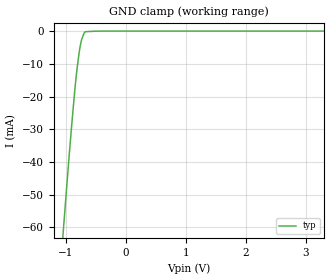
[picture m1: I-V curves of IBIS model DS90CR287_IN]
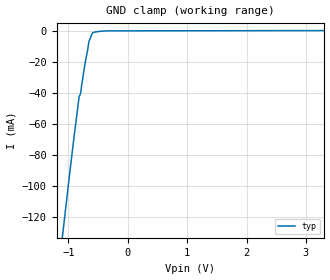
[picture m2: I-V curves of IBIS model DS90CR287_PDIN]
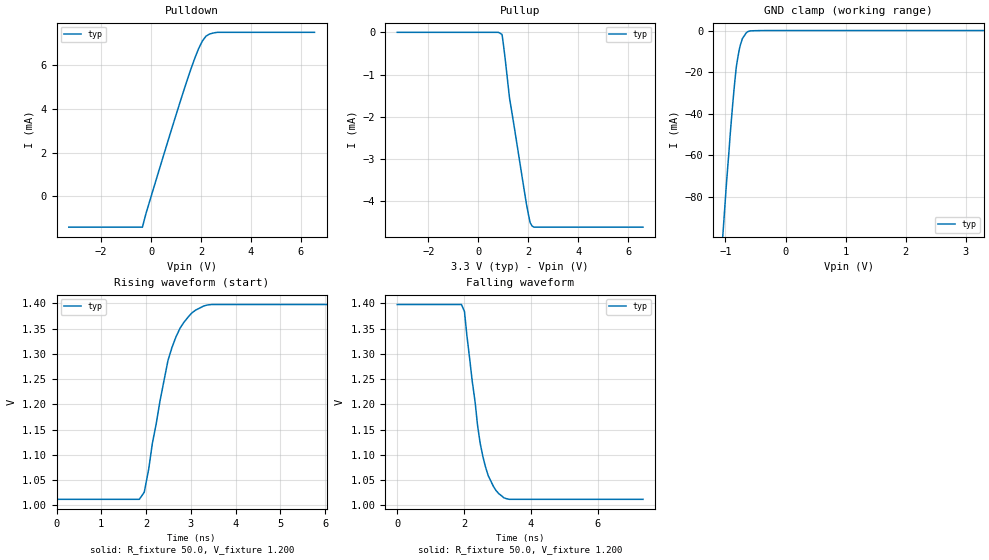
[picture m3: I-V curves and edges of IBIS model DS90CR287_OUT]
|   National Semiconductor Corporation
|   Interface Products Group
|   IBIS Model of DS90CR287MTD
|   High Speed Link Transmitter
|   56L TSSOP
[IBIS Ver]   3.2
[Comment char]  |_char
[File name]   ds90cr287.ibs
[File Rev]   1.4
[Date]   9/26/03
[Source]   File originated at National Semiconductor Corporation.
   Interface Group/Analog Division. All data based on
   Empirical Measurements(Bench).
[Notes]   File created by DT.
   Revision 1.0: The original model.
   Revision 1.1: Modified driver output pulldown
   and pullup to ensure no double
   counting of clamp current.
   Revision 1.2: Corrected ground and power clamp data.
   Revision 1.3: Changed Vdiff from .1 to 0 in pin mapping
   Changed Vref from 0 to 1.2 in V/T data
   Commented out c_fixutre in V/T data
   Revision 1.4: Modified pullup, pulldown,
   rising and falling waveform data;
[Disclaimer]
(C) Copyright National Semiconductor Corporation 2000
   All rights reserved
   National Semiconductor Corporation hereby grants
the user of this IBIS model a non-exclusive, nontransferable
license to use this IBIS model under the following terms.
Before using this IBIS model, the user should read this
license.  If the user does not accept these terms, the
IBIS model should be returned to National within 30 days.
   The user is granted this license only to use the
IBIS model and is not granted rights to sell, load, rent,
lease or license the IBIS model in whole or in part, or in
modified form to anyone other than user. User may modify
the IBIS model to suit its specific applications but rights
to derivative works and such modifications shall belong to
National.
   This IBIS model is provided on an "AS IS" basis and
National makes absolutely no warranty with respect to the
information contained herein. NATIONAL DISCLAIMS AND CUSTOMER
WAIVES ALL WARRANTIES, EXPRESS OR IMPLIED, INCLUDING
WARRANTIES OF MERCHANTABILITY OR FITNESS FOR A PARTICULAR
PURPOSE. The entire risk as to quality and performance is
with the Customer. ACCORDINGLY, IN NO EVENT SHALL THE
COMPANY BE LIABLE FOR ANY DAMAGES, WHETHER IN CONTRACT OR
TORT,INCLUDING ANY LOST PROFITS OR OTHER INCIDENTAL,
CONSEQUENTIAL, EXEMPLARY, OR PUNITIVE DAMAGES ARISING OUT
OF THE USE OR APPLICATION OF THE IBIS model provided in
this package. Further, National reserves the right to make
changes without notice to any product herein to improve
reliability, function, or design. National does not convey
any license under patent rights or any other intellectual
property rights, including those of third parties.
   National is not obligated to provide maintenance or support
for the licensed IBIS model.
Contact National at ATTN:INTERFACE APPLICATIONS/IBIS MODELS.
2900 Semiconductor Drive, M/S A2595, Santa Clara, CA 95052-8090
[Copyright]   Copyright 2000, National Semiconductor, All Rights Reserved
[Component]   DS90CR287MTD
[Manufacturer]  National Semiconductor Corp
[Package]
|   typ   min   max
R_pkg   61.4m   NA   NA
L_pkg   1.758nH   NA   NA
C_pkg   0.075pF   NA   NA
[Pin]   signal_name   model_name   R_pin   L_pin   C_pin
1   VCC   POWER   90.0m   3.077n   0.122p
2   TxIN5   DS90CR287_IN   90.0m   2.704n   0.107p
3   TxIN6   DS90CR287_IN   90.0m   2.405n   0.106p
4   TxIN7   DS90CR287_IN   70.0m   2.105n   0.096p
5   GND   GND   70.0m   1.874n   0.080p
6   TxIN8   DS90CR287_IN   60.0m   1.619n   0.071p
7   TxIN9   DS90CR287_IN   60.0m   1.414n   0.068p
8   TxIN10   DS90CR287_IN   60.0m   1.405n   0.068p
9   Vcc   POWER   50.0m   1.407n   0.055p
10   TxIN11   DS90CR287_IN   50.0m   1.396n   0.055p
11   TxIN12   DS90CR287_IN   50.0m   1.365n   0.055p
12   TxIN13   DS90CR287_IN   50.0m   1.318n   0.055p
13   GND   GND   40.0m   1.277n   0.057p
14   TxIN14   DS90CR287_IN   30.0m   1.249n   0.061p
15   TxIN15   DS90CR287_IN   30.0m   1.249n   0.061p
16   TxIN16   DS90CR287_IN   40.0m   1.277n   0.057p
17   Vcc   POWER   50.0m   1.318n   0.055p
18   TxIN17   DS90CR287_IN   50.0m   1.365n   0.055p
19   TxIN18   DS90CR287_IN   50.0m   1.396n   0.055p
20   TxIN19   DS90CR287_IN   50.0m   1.407n   0.055p
21   GND   GND   60.0m   1.405n   0.068p
22   TxIN20   DS90CR287_IN   60.0m   1.414n   0.068p
23   TxIN21   DS90CR287_IN   60.0m   1.619n   0.071p
24   TxIN22   DS90CR287_IN   70.0m   1.874n   0.080p
25   TxIN23   DS90CR287_IN   70.0m   2.105n   0.096p
26   Vcc   POWER   90.0m   2.405n   0.106p
27   TxIN24   DS90CR287_IN   90.0m   2.704n   0.107p
28   TxIN25   DS90CR287_IN   90.0m   3.077n   0.122p
29   GND   GND   90.0m   3.077n   0.122p
30   TxIN26   DS90CR287_IN   90.0m   2.704n   0.107p
31   TxCLKIN   DS90CR287_IN   90.0m   2.405n   0.106p
32   PWRDWN*   DS90CR287_PDIN   70.0m   2.105n   0.096p
33   PLLGND   GND   70.0m   1.874n   0.080p
34   PLLVCC   POWER   60.0m   1.619n   0.071p
35   PLLGND   GND   60.0m   1.414n   0.068p
36   LVDSGND   GND   60.0m   1.405n   0.068p
37   TxOUT3+   DS90CR287_OUT   50.0m   1.407n   0.055p
38   TxOUT3-   DS90CR287_OUT   50.0m   1.396n   0.055p
39   TxCLKOUT   DS90CR287_OUT   50.0m   1.365n   0.055p
40   TxCLKOUT   DS90CR287_OUT   50.0m   1.318n   0.055p
41   TxOUT2+   DS90CR287_OUT   40.0m   1.277n   0.057p
42   TxOUT2-   DS90CR287_OUT   30.0m   1.249n   0.061p
43   LVDSGND   GND   30.0m   1.249n   0.061p
44   LVDSVCC   POWER   40.0m   1.277n   0.057p
45   TxOUT1+   DS90CR287_OUT   50.0m   1.318n   0.055p
46   TxOUT1-   DS90CR287_OUT   50.0m   1.365n   0.055p
47   TxOUT0+   DS90CR287_OUT   50.0m   1.396n   0.055p
48   TxOUT0-   DS90CR287_OUT   50.0m   1.407n   0.055p
49   LVDSGND   GND   60.0m   1.405n   0.068p
50   TxIN27   DS90CR287_IN   60.0m   1.414n   0.068p
51   TxIN0   DS90CR287_IN   60.0m   1.619n   0.071p
52   TxIN1   DS90CR287_IN   70.0m   1.874n   0.080p
53   GND   GND   70.0m   2.105n   0.096p
54   TxIN2   DS90CR287_IN   90.0m   2.405n   0.106p
55   TxIN3   DS90CR287_IN   90.0m   2.704n   0.107p
56   TxIN4   DS90CR287_IN   90.0m   3.077n   0.122p
[Diff_pin]   inv_pin   vdiff   tdelay_typ   tdelay_min   tdelay_max
| The '+' pin is Diff_pin and the '-' pin is the inv_pin
37   38   0.0   0   0   0
39   40   0.0   0   0   0
41   42   0.0   0   0   0
45   46   0.0   0   0   0
47   48   0.0   0   0   0
| Models and submodels in the file (3): DS90CR287_IN (Input), DS90CR287_PDIN (Input), DS90CR287_OUT (3-state)
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|   Driver Input  MODEL
[Model]   DS90CR287_IN
Model_type   Input
|Signals   TxIN0 ~ TxIN27
Vinh = 2.0
Vinl = 0.8
|   typ   min   max
C_comp   5.910pF   NA   NA
|   typ   min   max
[Temperature Range]   25.0   NA   NA
[Voltage range]   3.3V   3.0V   3.6V
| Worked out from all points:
|   GND clamp passes 1 mA (typ) near -0.70 V on its own axis
[Power_clamp]
| Note that the[POWER_clamp]voltage table is referenced to Vcc
| and is calculated using Vtable=Vcc - Vmeasured.
|Voltage   I(typ)   I(min)   I(max)
-3V       0A         NA         NA
3V        0A         NA         NA
[GND_clamp]
|Voltage   I(typ)   I(min)   I(max)
-3.3V     -594.1mA   NA         NA
-1.001V   -51.39mA   NA         NA
-941.2mV  -37.29mA   NA         NA
-899.9mV  -28.27mA   NA         NA
-859.6mV  -19.87mA   NA         NA
-818.3mV  -12.37mA   NA         NA
-776.9mV  -6.424mA   NA         NA
-756.3mV  -4.202mA   NA         NA
-736.1mV  -2.573mA   NA         NA
-717mV    -1.615mA   NA         NA
-675.2mV  -194.8uA   NA         NA
3.3V      524nA      NA         NA
|   Driver PWRDWN* Input  MODEL
[Model]   DS90CR287_PDIN
Model_type   Input
|Signals   PWRDWN*
Vinh = 2.0
Vinl = 0.8
|   typ   min   max
C_comp   5.843pF   NA   NA
|   typ   min   max
[Temperature Range]   25.0   NA   NA
[Voltage range]   3.3V   3.0V   3.6V
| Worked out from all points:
|   GND clamp passes 1 mA (typ) near -0.57 V on its own axis
[Power_clamp]
| Note that the[POWER_clamp]voltage table is referenced to Vcc
| and is calculated using Vtable=Vcc - Vmeasured.
|Voltage   I(typ)   I(min)   I(max)
-3V       0A         NA         NA
3V        0A         NA         NA
[GND_clamp]
|Voltage   I(typ)   I(min)   I(max)
-3.3V     -863.2mA   NA         NA
-999.7mV  -98.78mA   NA         NA
-918.6mV  -72.42mA   NA         NA
-819.7mV  -42.41mA   NA         NA
-796.1mV  -40.44mA   NA         NA
-776.9mV  -35.09mA   NA         NA
-735.6mV  -24.85mA   NA         NA
-674.7mV  -11.91mA   NA         NA
-655mV    -6.957mA   NA         NA
-592.5mV  -1.248mA   NA         NA
-306.8mV  -9.428uA   NA         NA
3.3V      172.6uA    NA         NA
|   Driver Output  MODEL
[Model]   DS90CR287_OUT
Model_type   3-state
| Signals   TxOUT0 ~ TxOUT3; TxCLKOUT
Vmeas = 1.2V   |This is 0.0v differential on output
Cref = 5pF   |Timing specification test load capacitance value
Rref = 50   |Note: 100 Ohm between the two driver outputs
Vref = 1.2   |Timing specification test load voltage; GND
| variable   typ   min   max
C_comp   6.704pF   NA   NA
|   typ   min   max
[Temperature Range]   25.0   NA   NA
[Voltage range]   3.3V   3.0V   3.6V
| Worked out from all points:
|   slope of the pulldown table from 0 to 0.495 V, typ, clamps not added: 266 ohm
|   GND clamp passes 1 mA (typ) near -0.65 V on its own axis
|   rising waveform, R_fixture 50.0, V_fixture 1.200: 20-80 % time 526ps typ, NA min, NA max; typ from 1.01 V to 1.4 V
|   falling waveform, R_fixture 50.0, V_fixture 1.200: 20-80 % time 479ps typ, NA min, NA max; typ from 1.4 V to 1.01 V
[Pulldown]
| Voltage   I(typ)   I(min)   I(max)
-3.3V     -1.408mA   NA         NA
-350mV    -1.408mA   NA         NA
-200mV    -758uA     NA         NA
475mV     1.786mA    NA         NA
1.45V     5.331mA    NA         NA
1.75V     6.312mA    NA         NA
1.9V      6.74mA     NA         NA
2.05V     7.09mA     NA         NA
2.2V      7.321mA    NA         NA
2.35V     7.422mA    NA         NA
2.65V     7.496mA    NA         NA
6.55V     7.496mA    NA         NA
[Pullup]
| Note that the[Pullup]voltage table is referenced to Vcc
| and is calculated using Vtable=Vcc - Vmeasured.
|Voltage   I(typ)   I(min)   I(max)
-3.25V    0A         NA         NA
800mV     -600nA     NA         NA
950mV     -51.4uA    NA         NA
1.025V    -380.3uA   NA         NA
1.1V      -755.3uA   NA         NA
1.25V     -1.556mA   NA         NA
1.4V      -2.095mA   NA         NA
1.925V    -4.051mA   NA         NA
2.075V    -4.497mA   NA         NA
2.15V     -4.577mA   NA         NA
2.225V    -4.607mA   NA         NA
6.6V      -4.607mA   NA         NA
[GND_clamp]
| Outputs in Tri-state.
| Voltage   I(typ)   I(min)   I(max)
-3.3V     -1.034A    NA         NA
-1.001V   -81.02mA   NA         NA
-983mV    -73.48mA   NA         NA
-921.5mV  -50.22mA   NA         NA
-900.9mV  -42.95mA   NA         NA
-859.6mV  -29.11mA   NA         NA
-819.2mV  -17.54mA   NA         NA
-767.2mV  -8.785mA   NA         NA
-719.4mV  -3.945mA   NA         NA
-634.3mV  -657.5uA   NA         NA
-347.7mV  -11.87uA   NA         NA
3.3V      524nA      NA         NA
[POWER_clamp]
| Note that the[POWER_clamp]voltage table is referenced to Vcc
| and is calculated using Vtable=Vcc - Vmeasured.
| Outputs in Tri-state.
|Voltage   I(typ)   I(min)   I(max)
-3V       0A         NA         NA
3V        0A         NA         NA
[Ramp]
| Note: Ramp rate measured on single-ended Driver Output.
|   typ   min   max
dV/dt_r   204.0m/446.03p   NA   NA
dV/dt_f   205.5m/372.29p   NA   NA
R_load = 100Ohm | Note: This 100 Ohm is across the two driver output
[Rising Waveform]
R_fixture = 50.0
V_fixture = 1.200
V_fixture_min=1.20
V_fixture_max=1.21
|C_fixture = 8.0pF
|Time   V(typ)   V(min)  V(max)
0s        1.012V     NA         NA
1.85ns    1.012V     NA         NA
1.96ns    1.026V     NA         NA
2.06ns    1.072V     NA         NA
2.31ns    1.206V     NA         NA
2.49ns    1.287V     NA         NA
2.76ns    1.351V     NA         NA
3.11ns    1.387V     NA         NA
3.47ns    1.398V     NA         NA
8.17ns    1.398V     NA         NA
[Falling Waveform]
R_fixture = 50.0
V_fixture = 1.200
V_fixture_min=1.20
V_fixture_max=1.21
|C_fixture = 8.0pF
|Time   V(typ)   V(min)  V(max)
0s        1.398V     NA         NA
1.92ns    1.398V     NA         NA
2.01ns    1.384V     NA         NA
2.08ns    1.338V     NA         NA
2.4ns     1.159V     NA         NA
2.56ns    1.097V     NA         NA
2.72ns    1.059V     NA         NA
2.88ns    1.037V     NA         NA
3.19ns    1.015V     NA         NA
7.35ns    1.012V     NA         NA
